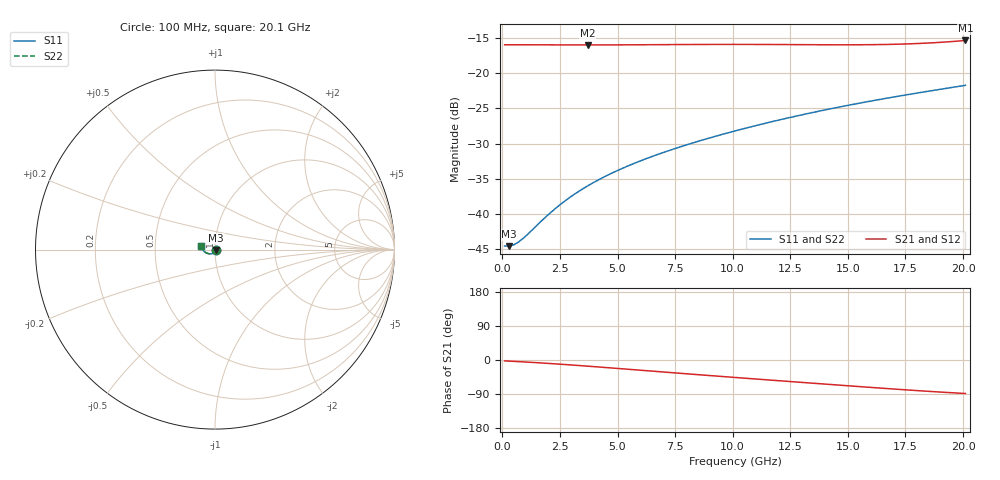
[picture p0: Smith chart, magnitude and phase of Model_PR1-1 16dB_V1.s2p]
!version-1
!date-07.2020
!Series
#	GHZ S RI R 50.0
!	FREQ.GHZ	S11RE	S11IM	S21RE	S21IM	S12RE	S12IM	S22RE	S22IM
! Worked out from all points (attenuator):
!   101 points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, 100 MHz to 20.1 GHz, reference 50 ohm
!   highest |S21| = -15.30 dB at 20.1 GHz (marker M1); lowest = -15.9 dB at 3.7 GHz (marker M2)
!   lowest |S11| = -44.6 dB at 300 MHz (marker M3), VSWR 1.01, Z = 50.5 - j0.233 ohm
!   |S11| at or under -10 dB: start of sweep to end of sweep
!   |S22| runs from -44.6 to -21.7 dB; largest |S21 - S12| = 0
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0.1  0.00573 -0.00133  0.16 -0.00671  0.16 -0.00671  0.00573 -0.00133
0.3  0.00539 -0.0023  0.1599 -0.00837  0.1599 -0.00837  0.00539 -0.0023
0.5  0.00504 -0.00326  0.1598 -0.0101  0.1598 -0.0101  0.00504 -0.00326
0.7  0.00466 -0.00419  0.1597 -0.0119  0.1597 -0.0119  0.00466 -0.00419
1.1  0.00386 -0.00598  0.1593 -0.0157  0.1593 -0.0157  0.00386 -0.00598
1.9  0.00205 -0.0093  0.1581 -0.0239  0.1581 -0.0239  0.00205 -0.0093
2.3  0.00103 -0.0108  0.1573 -0.0284  0.1573 -0.0284  0.00103 -0.0108
2.9  -0.000619 -0.0129  0.1559 -0.0352  0.1559 -0.0352  -0.000619 -0.0129
3.5  -0.00243 -0.0149  0.154 -0.0423  0.154 -0.0423  -0.00243 -0.0149
3.7  -0.00306 -0.0155  0.1534 -0.0447  0.1534 -0.0447  -0.00306 -0.0155
4.3  -0.00508 -0.0171  0.1511 -0.052  0.1511 -0.052  -0.00508 -0.0171
5.1  -0.00799 -0.019  0.1475 -0.0617  0.1475 -0.0617  -0.00799 -0.019
5.9  -0.0112 -0.0206  0.1433 -0.0714  0.1433 -0.0714  -0.0112 -0.0206
6.9  -0.0154 -0.0221  0.1372 -0.0831  0.1372 -0.0831  -0.0154 -0.0221
8.3  -0.022 -0.0233  0.1271 -0.0986  0.1271 -0.0986  -0.022 -0.0233
10.1  -0.0311 -0.0233  0.1117 -0.116  0.1117 -0.116  -0.0311 -0.0233
11.7  -0.0398 -0.0216  0.0961 -0.1289  0.0961 -0.1289  -0.0398 -0.0216
13.5  -0.0497 -0.0177  0.0769 -0.1406  0.0769 -0.1406  -0.0497 -0.0177
15.1  -0.0583 -0.0123  0.0589 -0.1488  0.0589 -0.1488  -0.0583 -0.0123
16.9  -0.0674 -0.00372  0.0385 -0.1566  0.0385 -0.1566  -0.0674 -0.00372
18.5  -0.0744 0.00639  0.021 -0.1635  0.021 -0.1635  -0.0744 0.00639
20.1  -0.08 0.0192  0.00493 -0.1718  0.00493 -0.1718  -0.08 0.0192
